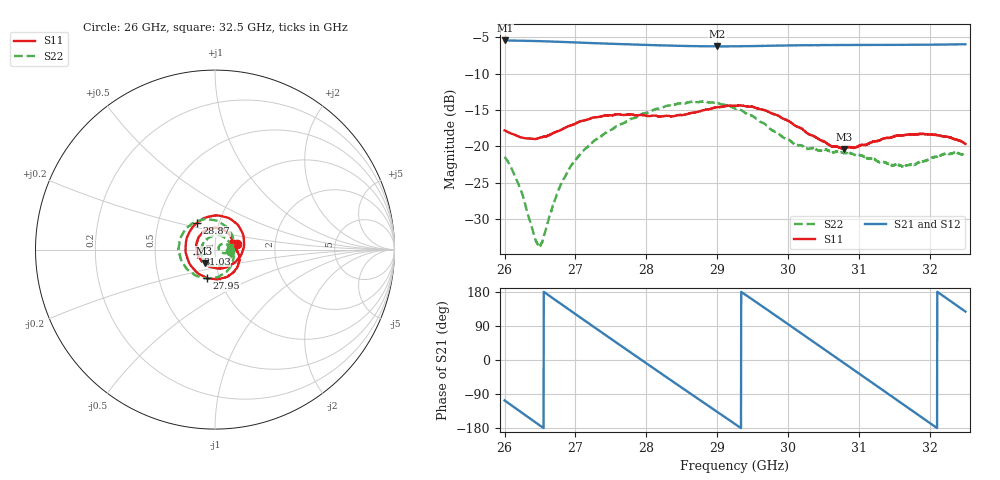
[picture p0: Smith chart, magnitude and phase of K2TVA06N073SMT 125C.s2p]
!Keysight Technologies,N5247B,US57180393,A.17.35.14
!Date: Thursday, May 08, 2025 10:36:17
!Correction: S11(C  2-Port  )
!S21(C  2-Port  )
!S12(C  2-Port  )
!S22(C  2-Port  )
!S2P File: Measurements: S11, S21, S12, S22:
# Hz S  RI  R 50
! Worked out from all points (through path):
!   2001 points, 26 GHz to 32.5 GHz, reference 50 ohm
!   highest |S21| = -5.41 dB at 26.01 GHz (marker M1); lowest = -6.2 dB at 29 GHz (marker M2)
!   group delay of S21, straight-line fit = 360 ps
!   lowest |S11| = -20.4 dB at 30.79 GHz (marker M3), VSWR 1.21, Z = 44 - j6.78 ohm
!   |S11| at or under -10 dB: start of sweep to end of sweep
!   |S22| runs from -33.8 to -13.8 dB; largest |S21 - S12| = 0.0016
!   S11 on the Smith chart (normalised r, x): 26 GHz: 1.28, +0.08; 27.95 GHz: 0.87, -0.28; 28.87 GHz: 0.79, +0.24; 31.03 GHz: 0.82, -0.04; 32.5 GHz: 1.21, +0.09
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2.6e10  0.1246 0.0321  -0.1543 -0.5135  -0.1546 -0.5133  0.0842 -0.0082
2.60065e10  0.1242 0.0313  -0.162 -0.5114  -0.1624 -0.511  0.0834 -0.00895
2.649075e10  0.1143 0.0028  -0.5251 -0.0743  -0.5253 -0.0741  0.02 0.00478
2.6767e10  0.1269 -0.0149  -0.4618 0.2497  -0.4618 0.2499  0.0399 0.0312
2.70855e10  0.1355 -0.0625  -0.1761 0.487  -0.1761 0.4871  0.09 0.00828
2.74625e10  0.0956 -0.1324  0.2487 0.4447  0.2492 0.4449  0.0916 -0.0881
2.795325e10  -0.0442 -0.158  0.4999 -0.0237  0.5001 -0.0244  -0.0488 -0.1609
2.816775e10  -0.1108 -0.1163  0.4288 -0.2514  0.4288 -0.2514  -0.1193 -0.1372
2.85285e10  -0.1635 0.0192  0.1127 -0.4786  0.1126 -0.479  -0.1941 -0.0388
2.8873e10  -0.0992 0.1498  -0.2496 -0.4202  -0.2498 -0.4198  -0.1851 0.0793
2.9003e10  -0.0521 0.1785  -0.3593 -0.33  -0.3596 -0.3305  -0.1595 0.1185
2.925e10  0.0486 0.1841  -0.48 -0.0936  -0.4801 -0.0932  -0.0807 0.163
2.95425e10  0.1369 0.123  -0.4399 0.2187  -0.4398 0.2189  0.0233 0.154
2.9861e10  0.1614 0.0185  -0.1879 0.4571  -0.1884 0.4576  0.0989 0.0718
3.03355e10  0.0714 -0.095  0.3149 0.3849  0.3156 0.3849  0.0728 -0.0644
3.078725e10  -0.058 -0.0763  0.4941 -0.0707  0.4935 -0.0706  -0.0232 -0.0869
3.102775e10  -0.0992 -0.0221  0.3851 -0.3173  0.3853 -0.3181  -0.0626 -0.0594
3.141775e10  -0.083 0.0782  -0.00323 -0.5006  -0.00317 -0.5001  -0.0738 0.0155
3.1681e10  -0.0319 0.1163  -0.2855 -0.4111  -0.2859 -0.4113  -0.041 0.0616
3.199625e10  0.038 0.1144  -0.4867 -0.1212  -0.4867 -0.1206  0.0238 0.0787
3.223675e10  0.0797 0.0847  -0.4799 0.1517  -0.4796 0.1523  0.0665 0.0586
3.25e10  0.0978 0.0349  -0.3098 0.3988  -0.3095 0.3992  0.0856 0.015
